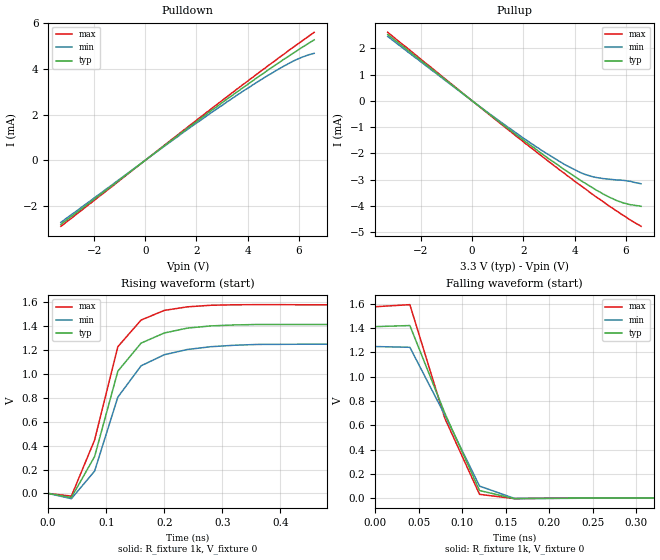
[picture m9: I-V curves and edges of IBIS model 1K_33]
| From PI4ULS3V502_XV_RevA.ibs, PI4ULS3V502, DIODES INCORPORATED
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[Model]   1K_33
Model_type  Output
Vref = 0
Rref = 10k
Vmeas = 1.65
C_comp   8.864pF   8.757pF   8.982pF
[Voltage Range]   3.30V   3.0V   3.6V
[Temperature Range]   25   85   -40
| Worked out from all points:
|   slope of the pulldown table from 0 to 0.495 V, typ, clamps not added: 1.17 kohm
|   slope of the pullup table from 0 to 0.495 V, typ, clamps not added: 1.32 kohm
|   rising waveform, R_fixture 1k, V_fixture 0: 20-80 % time 61.3ps typ, 65.3ps min, 57.4ps max; typ from 0 V to 1.41 V
|   falling waveform, R_fixture 1k, V_fixture 0: 20-80 % time 50ps typ, 52.2ps min, 47.7ps max; typ from 1.41 V to 0 V
[Pullup]
-3.3V     2.52mA     2.45mA     2.61mA
1.4V      -1.05mA    -1.01mA    -1.1mA
2.7V      -2mA       -1.88mA    -2.09mA
3.6V      -2.62mA    -2.42mA    -2.76mA
4.4V      -3.13mA    -2.8mA     -3.34mA
4.9V      -3.43mA    -2.93mA    -3.7mA
5.4V      -3.69mA    -2.99mA    -4.04mA
5.9V      -3.89mA    -3.03mA    -4.36mA
6.6V      -4.02mA    -3.16mA    -4.78mA
[Pulldown]
-3.3V     -2.81mA    -2.72mA    -2.89mA
1.4V      1.19mA     1.15mA     1.23mA
3.8V      3.16mA     3.01mA     3.3mA
4.8V      3.95mA     3.72mA     4.14mA
5.8V      4.7mA      4.35mA     4.96mA
6.1V      4.92mA     4.5mA      5.2mA
6.6V      5.27mA     4.68mA     5.6mA
[Rising Waveform]
R_fixture =   1k
C_fixture =   0
L_fixture =   0
V_fixture =   0
V_fixture_min = 0
V_fixture_max = 0
|   Time   V(typ)   V(min)   V(max)
0s        0V         0V         0V
40ps      -34.58mV   -44.09mV   -22.45mV
80ps      308.3mV    186.7mV    446.9mV
120ps     1.023V     805.8mV    1.228V
160ps     1.258V     1.068V     1.451V
200ps     1.343V     1.161V     1.532V
240ps     1.384V     1.205V     1.562V
320ps     1.41V      1.24V      1.579V
440ps     1.414V     1.249V     1.579V
3.96ns    1.413V     1.248V     1.578V
[Falling Waveform]
R_fixture =   1k
C_fixture =   0
L_fixture =   0
V_fixture =   0
V_fixture_min = 0
V_fixture_max = 0
|   Time   V(typ)   V(min)   V(max)
0s        1.412V     1.248V     1.576V
40ps      1.421V     1.242V     1.593V
80ps      701.5mV    686mV      659.5mV
120ps     62.27mV    98.65mV    30.72mV
160ps     -4.929mV   -2.533mV   -4.275mV
320ps     178.3uV    215.6uV    142.1uV
3.96ns    0V         0V         0V
[Ramp]
| variable   typ   min   max
dV/dt_r   0.9/55.1E-09   0.9/61.0E-09   0.9/51.2E-09
dV/dt_f   0.9/38.0E-09   0.9/42.6E-09   0.9/35.2E-09
R_load = 1k
| End component PI4ULS3V504
